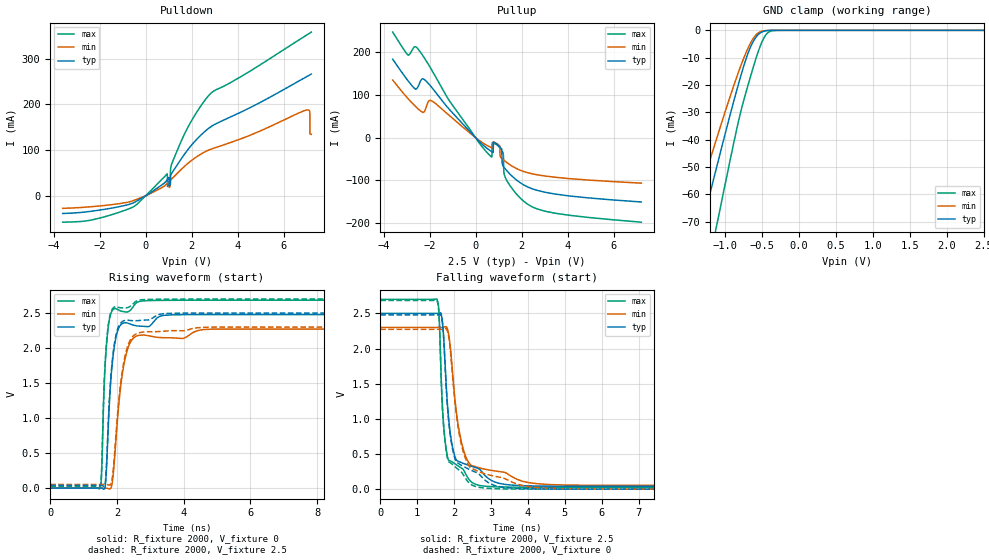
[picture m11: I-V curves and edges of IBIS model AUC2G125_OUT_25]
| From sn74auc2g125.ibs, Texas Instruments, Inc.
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[Model]   AUC2G125_OUT_25
Model_type  3-state
Enable   Active-Low
Vref =   0
Rref =   500
Cref =   30p
Vmeas =   1.25
| variable   typ   min   max
C_comp   4.95pF   4.40pF   5.29pF
| C_pullup   6.35pF   0.05pF   11.30pF
| C_pulldown   6.36pF   5.05pF   15.82pF
| C_tri-state   4.95pF   4.40pF   5.29pF
[Temperature Range]   40   100   -40
| Ambient temperature   25   85   -40
[Voltage range]   2.5   2.3   2.7
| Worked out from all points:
|   slope of the pulldown table from 0 to 0.375 V, typ, clamps not added: 30.9 ohm
|   slope of the pullup table from 0 to 0.375 V, typ, clamps not added: 19.2 ohm
|   GND clamp passes 1 mA (typ) near -0.53 V on its own axis
|   rising waveform, R_fixture 2000, V_fixture 0: 20-80 % time 203ps typ, 297ps min, 144ps max; typ from 0 V to 2.48 V
|   falling waveform, R_fixture 2000, V_fixture 2.5: 20-80 % time 253ps typ, 362ps min, 172ps max; typ from 2.5 V to 0.04 V
|   rising waveform, R_fixture 2000, V_fixture 2.5: 20-80 % time 203ps typ, 297ps min, 143ps max; typ from 0.04 V to 2.5 V
|   falling waveform, R_fixture 2000, V_fixture 0: 20-80 % time 257ps typ, 369ps min, 172ps max; typ from 2.48 V to 0 V
[GND Clamp]
| AUC2G125_OUT_25
|   Voltage   I(typ)   I(min)   I(max)
-3.6V     -324.8mA   -272.6mA   -395.3mA
-1.515V   -93.62mA   -75.35mA   -124.4mA
-1.455V   -87.03mA   -69.89mA   -116.5mA
-1.295V   -69.56mA   -55.5mA    -95.38mA
-1.105V   -49.1mA    -38.82mA   -70.28mA
-850mV    -22.72mA   -17.71mA   -37.11mA
-725mV    -11.19mA   -8.712mA   -23.46mA
-625mV    -4.389mA   -3.231mA   -14.1mA
-525mV    -974.6uA   -541.7uA   -5.852mA
-435mV    -119.5uA   -65.92uA   -1.256mA
-325mV    -4.911uA   -4.228uA   -43.96uA
2.5V      725.8pA    178.4nA    1.045nA
[Pulldown]
| AUC2G125_OUT_25
|   Voltage   I(typ)   I(min)   I(max)
-3.6V     -38.75mA   -27.46mA   -57.79mA
-580mV    -16.57mA   -11.5mA    -25.48mA
935mV     34.57mA    26.63mA    48.15mA
950mV     35.58mA    27.35mA    20.2mA
1.075V    24.55mA    33.22mA    46.33mA
1.62V     85.87mA    61.08mA    127.6mA
2.775V    148.9mA    100.6mA    221.1mA
7.005V    260.8mA    187.6mA    351.9mA
7.13V     264.4mA    184.5mA    355.9mA
7.135V    264.5mA    182.7mA    356mA
7.14V     264.6mA    135.1mA    356.2mA
7.2V      266.3mA    134.5mA    358.1mA
[Pullup]
| AUC2G125_OUT_25
|   Voltage   I(typ)   I(min)   I(max)
-3.6V     183.4mA    134.7mA    246.6mA
-2.935V   133mA      91.26mA    193mA
-2.48V    121.4mA    66.42mA    205.9mA
-1.895V   116.7mA    85.53mA    157.1mA
505mV     -25.26mA   -18.37mA   -35.17mA
1.03V     -20.52mA   -18.17mA   -22.58mA
1.14V     -26.75mA   -48.47mA   -30.66mA
1.2V      -66.47mA   -51.27mA   -36.41mA
1.23V     -69.04mA   -52.63mA   -81.1mA
1.32V     -74.92mA   -56.52mA   -96.36mA
2.17V     -112.6mA   -80.39mA   -151.9mA
7.2V      -150.3mA   -106.2mA   -197.4mA
[Ramp]
| AUC2G125_OUT_25
| variable   typ   min   max
dV/dt_r   1.50/2.04E-10   1.37/2.99E-10   1.62/1.44E-10
dV/dt_f   1.48/2.54E-10   1.35/3.63E-10   1.61/1.73E-10
R_load = 2000
[Rising Waveform]
| AUC2G125_OUT_25
R_fixture =   2000
C_fixture =   0
L_fixture =   0
V_fixture =   0
V_fixture_min = 0
V_fixture_max = 0
|   Time   V(typ)   V(min)   V(max)
0s        11.11nV    33.4nV     1.993nV
1.505ns   609.1uV    70.82uV    10.19mV
1.54ns    -705.4uV   159.6uV    233.2mV
1.655ns   59.3mV     -265.9uV   1.839V
1.78ns    1.284V     -11.15mV   2.424V
1.865ns   1.811V     101.7mV    2.541V
1.955ns   2.12V      595.7mV    2.564V
2.215ns   2.361V     1.783V     2.519V
2.665ns   2.314V     2.183V     2.665V
20ns      2.479V     2.273V     2.683V
[Falling Waveform]
| AUC2G125_OUT_25
R_fixture =   2000
C_fixture =   0
L_fixture =   0
V_fixture =   2.5
V_fixture_min = 2.3
V_fixture_max = 2.7
|   Time   V(typ)   V(min)   V(max)
0s        2.5V       2.3V       2.7V
1.535ns   2.5V       2.3V       2.704V
1.595ns   2.502V     2.299V     2.451V
1.68ns    2.4V       2.3V       1.209V
1.825ns   1.17V      2.269V     451.1mV
1.98ns    546mV      1.521V     377.4mV
2.185ns   381mV      701.5mV    304.3mV
2.66ns    292.7mV    307.3mV    57.22mV
3.985ns   47.43mV    96.41mV    27.32mV
20ns      40.45mV    53.08mV    26.22mV
[Rising Waveform]
| AUC2G125_OUT_25
R_fixture =   2000
C_fixture =   0
L_fixture =   0
V_fixture =   2.5
V_fixture_min = 2.3
V_fixture_max = 2.7
|   Time   V(typ)   V(min)   V(max)
0s        40.42mV    53.07mV    26.21mV
1.505ns   41.02mV    53.14mV    36.78mV
1.54ns    39.72mV    53.23mV    264.6mV
1.63ns    34.16mV    53.58mV    1.646V
1.685ns   332.2mV    51.46mV    2.068V
1.8ns     1.478V     47.42mV    2.486V
1.935ns   2.098V     539mV      2.588V
2.245ns   2.396V     1.894V     2.575V
2.72ns    2.397V     2.225V     2.689V
20ns      2.5V       2.3V       2.7V
[Falling Waveform]
| AUC2G125_OUT_25
R_fixture =   2000
C_fixture =   0
L_fixture =   0
V_fixture =   0
V_fixture_min = 0
V_fixture_max = 0
|   Time   V(typ)   V(min)   V(max)
0s        2.479V     2.273V     2.683V
1.535ns   2.478V     2.273V     2.687V
1.595ns   2.48V      2.273V     2.432V
1.68ns    2.376V     2.273V     1.19V
1.82ns    1.18V      2.247V     440.3mV
1.97ns    541.2mV    1.54V      344.7mV
2.175ns   347mV      690mV      253.6mV
2.61ns    235mV      263.2mV    33.51mV
4.77ns    1.451mV    8.61mV     284.1uV
20ns      27.56uV    4.219uV    11.82uV
